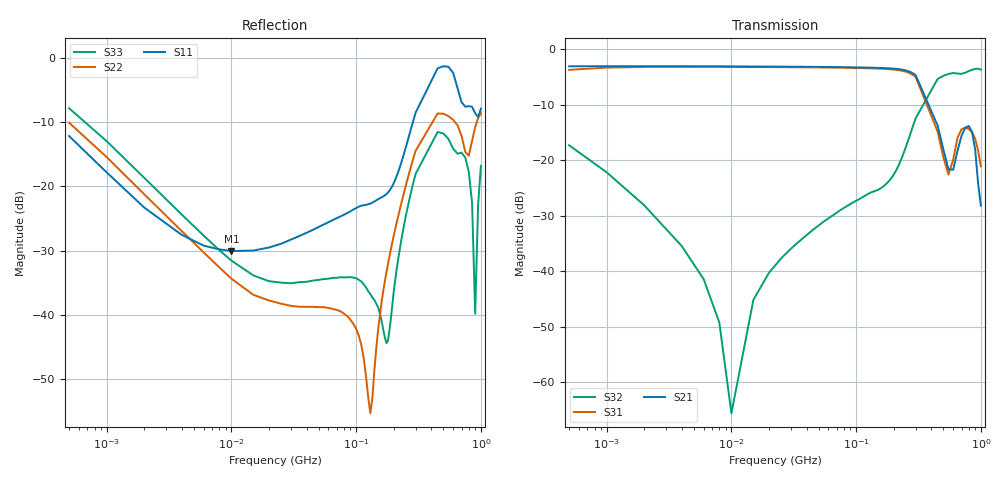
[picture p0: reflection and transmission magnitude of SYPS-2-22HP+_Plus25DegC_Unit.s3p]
!Created: 08-14-2018 at 12:36:30
!Mini-Circuits
!S3P DATA File Format
!Type: POWER SPLTR/CMBD
!MODEL: SYPS-2-22HP+
!S/N: Unit 1
!TEST CONDITIONS: Z:50 OHM SYSTEM, INPUT POWER = -10dBm, TEMP:25 degree C
!REMARK: Full 3 port calibration using Ecal. Port extension done.
# MHZ S DB R 50
!Frequency  S11 dB  S11 DEG  S12 dB  S12 DEG  S13 dB  S13 DEG
!  S21 dB  S21 DEG  S22 dB  S22 DEG  S23 dB  S23 DEG
!  S31 dB  S31 DEG  S32 dB  S32 DEG  S33 dB  S33 DEG
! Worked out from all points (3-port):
!   67 points, 500 kHz to 1 GHz, reference 50 ohm
!   strongest paths, dB at 500 kHz, 60 MHz, 145 MHz, 260 MHz, 1 GHz:
!     S21: -3.1, -3.2, -3.4, -4.0, -28.2
!     S31: -3.8, -3.3, -3.5, -4.2, -21.1
!     S32: -17.3, -30.5, -25.5, -16.6, -3.7
!   lowest |S11| = -30.1 dB at 10 MHz (marker M1), VSWR 1.06, Z = 52.4 + j2.16 ohm
!   |S11| at or under -10 dB: start of sweep to 285.4 MHz
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0.5  -12.20 99.9  -3.13 10.4  -3.76 16.4
     -3.12 10.2  -10.12 112.0  -17.34 -45.9
     -3.75 16.3  -17.33 -45.7  -7.88 116.7
6  -29.22 51.7  -3.12 -1.4  -3.20 -0.7
   -3.11 -1.4  -30.28 92.2  -41.57 -91.4
   -3.20 -0.7  -41.43 -91.7  -27.67 78.0
10  -30.05 40.8  -3.13 -3.1  -3.22 -2.7
    -3.13 -3.1  -34.35 91.3  -68.70 -0.4
    -3.22 -2.7  -65.56 -23.6  -31.55 69.1
25  -28.93 34.7  -3.17 -8.2  -3.27 -8.0
    -3.17 -8.2  -38.23 85.2  -37.60 74.2
    -3.27 -8.0  -37.70 73.5  -34.97 53.8
130  -22.68 -14.1  -3.36 -42.3  -3.48 -42.2
     -3.36 -42.3  -55.26 127.1  -25.83 80.7
     -3.48 -42.2  -25.87 80.6  -36.75 9.2
180  -20.97 -65.5  -3.47 -60.4  -3.62 -60.0
     -3.47 -60.4  -32.07 -163.7  -23.92 94.9
     -3.62 -60.0  -23.95 94.9  -43.99 -100.8
450  -1.68 69.9  -13.81 157.0  -14.88 167.2
     -13.77 156.9  -8.69 68.7  -5.40 63.1
     -14.85 167.0  -5.40 63.1  -11.57 55.2
800  -7.55 -45.9  -13.86 -31.9  -14.37 -112.0
     -13.85 -31.6  -15.25 27.7  -3.99 7.5
     -14.38 -111.5  -3.98 7.6  -17.77 -31.1
900  -8.67 -121.8  -18.08 -93.4  -16.17 -158.3
     -18.09 -93.0  -10.80 34.1  -3.61 -4.8
     -16.16 -157.6  -3.58 -4.8  -39.80 -6.5
1000  -7.95 111.8  -28.27 -74.1  -21.14 159.3
      -28.19 -73.3  -8.67 17.4  -3.72 -18.3
      -21.11 160.2  -3.69 -18.4  -16.82 72.1
